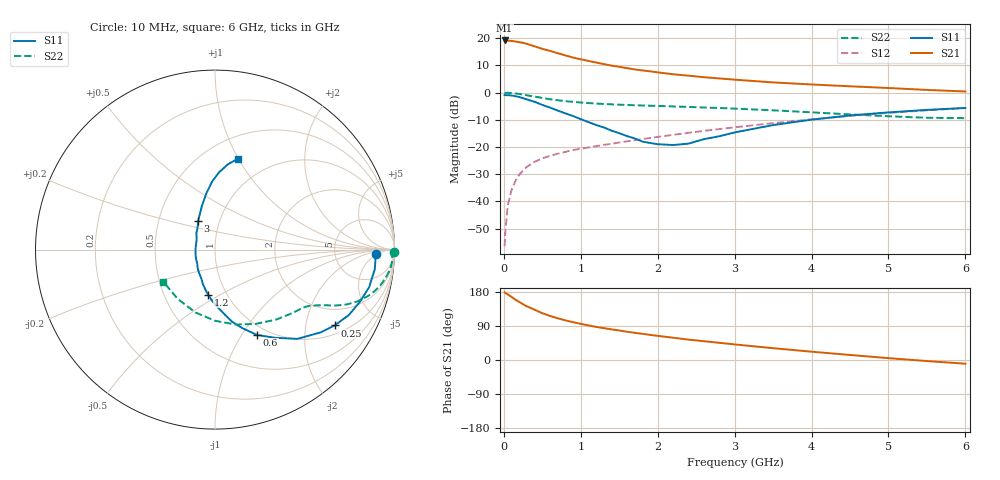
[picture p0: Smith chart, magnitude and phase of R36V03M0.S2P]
! SIEMENS Small Signal Semiconductors
! BFR181
! Si NPN RF Bipolar Junction Transistor in SOT23
! VCE = 6 V  IC = 3 mA
! Common Emitter S-Parameters:  May  1996
# GHz  S  MA  R  50
!  f  S11  S21  S12  S22
! GHz  MAG  ANG  MAG  ANG  MAG  ANG  MAG  ANG
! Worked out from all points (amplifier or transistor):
!   36 points, 10 MHz to 6 GHz, reference 50 ohm
!   highest |S21| = 19.2 dB at 10 MHz (marker M1)
!   |S21| within 3 dB of that: start of sweep to 490.7 MHz
!   unconditionally stable (mu >= 1): 1.398 GHz to 3.25 GHz
!   at 250 MHz: K = 0.30, MSG = 23.5 dB, |S12| = -28.7 dB
!   at 1.4 GHz: K = 1.00, MAG = 14.2 dB, |S12| = -18.8 dB
!   at 6 GHz: K = 0.86, MSG = 3.1 dB, |S12| = -5.7 dB
!   lowest NFmin = 1.40 dB at 450 MHz
!   S11 on the Smith chart (normalised r, x): 10 MHz: 18, -4; 250 MHz: 1.30, -2.91; 600 MHz: 0.88, -1.17; 1.2 GHz: 0.82, -0.44; 3 GHz: 0.79, +0.26; 6 GHz: 0.71, +0.99
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0.01  0.8998 -1.5  9.082 178.4  0.0015 96.4  0.9957 -0.7
0.02  0.896 -2.7  9.056 176.8  0.0028 92.8  0.9845 -1.3
0.05  0.8971 -7.0  8.982 173.1  0.0083 83.7  0.9907 -3.3
0.1  0.884 -13.7  8.912 166.7  0.0161 81.9  0.9825 -6.3
0.15  0.8576 -20.0  8.688 159.2  0.0238 77.8  0.9632 -9.6
0.25  0.7888 -32.4  8.214 147.1  0.0369 71.7  0.9188 -14.6
0.3  0.7475 -38.1  7.854 141.5  0.0433 69.8  0.8921 -16.8
0.4  0.6768 -47.3  7.073 132.7  0.0534 65.6  0.8427 -20.1
0.5  0.5933 -55.9  6.367 123.5  0.0617 62.5  0.797 -22.5
0.6  0.5298 -63.8  5.836 116.3  0.0689 60.8  0.7548 -24.3
0.7  0.466 -70.5  5.306 110.1  0.0752 59.7  0.7218 -25.6
0.8  0.4146 -76.5  4.816 104.6  0.0811 58.7  0.6945 -26.5
0.9  0.3702 -81.0  4.405 99.8  0.0877 58.3  0.675 -27.4
1.1  0.2862 -93.2  3.821 91.3  0.0979 58.2  0.6415 -29.0
1.2  0.2533 -98.8  3.57 87.4  0.1038 58.4  0.6285 -29.8
1.6  0.1587 -123.7  2.81 74.5  0.1269 59.3  0.5917 -32.9
2.2  0.1086 175.3  2.171 58.8  0.1671 59.3  0.5562 -39.5
3  0.185 120.6  1.727 41.1  0.2301 56.6  0.5065 -51.2
3.5  0.2527 106.9  1.538 31.2  0.2739 53.5  0.4716 -61.4
4.5  0.3798 92.4  1.304 13.3  0.372 44.4  0.3968 -89.9
5.5  0.4804 81.4  1.119 -2.8  0.4717 32.2  0.3442 -127.3
6  0.5218 75.9  1.048 -9.8  0.5181 25.2  0.3387 -148.1
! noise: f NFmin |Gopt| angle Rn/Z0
0.45  1.4  0.56  17  0.36
0.9  1.5  0.45  35  0.34
1.8  1.85  0.25  82  0.36
